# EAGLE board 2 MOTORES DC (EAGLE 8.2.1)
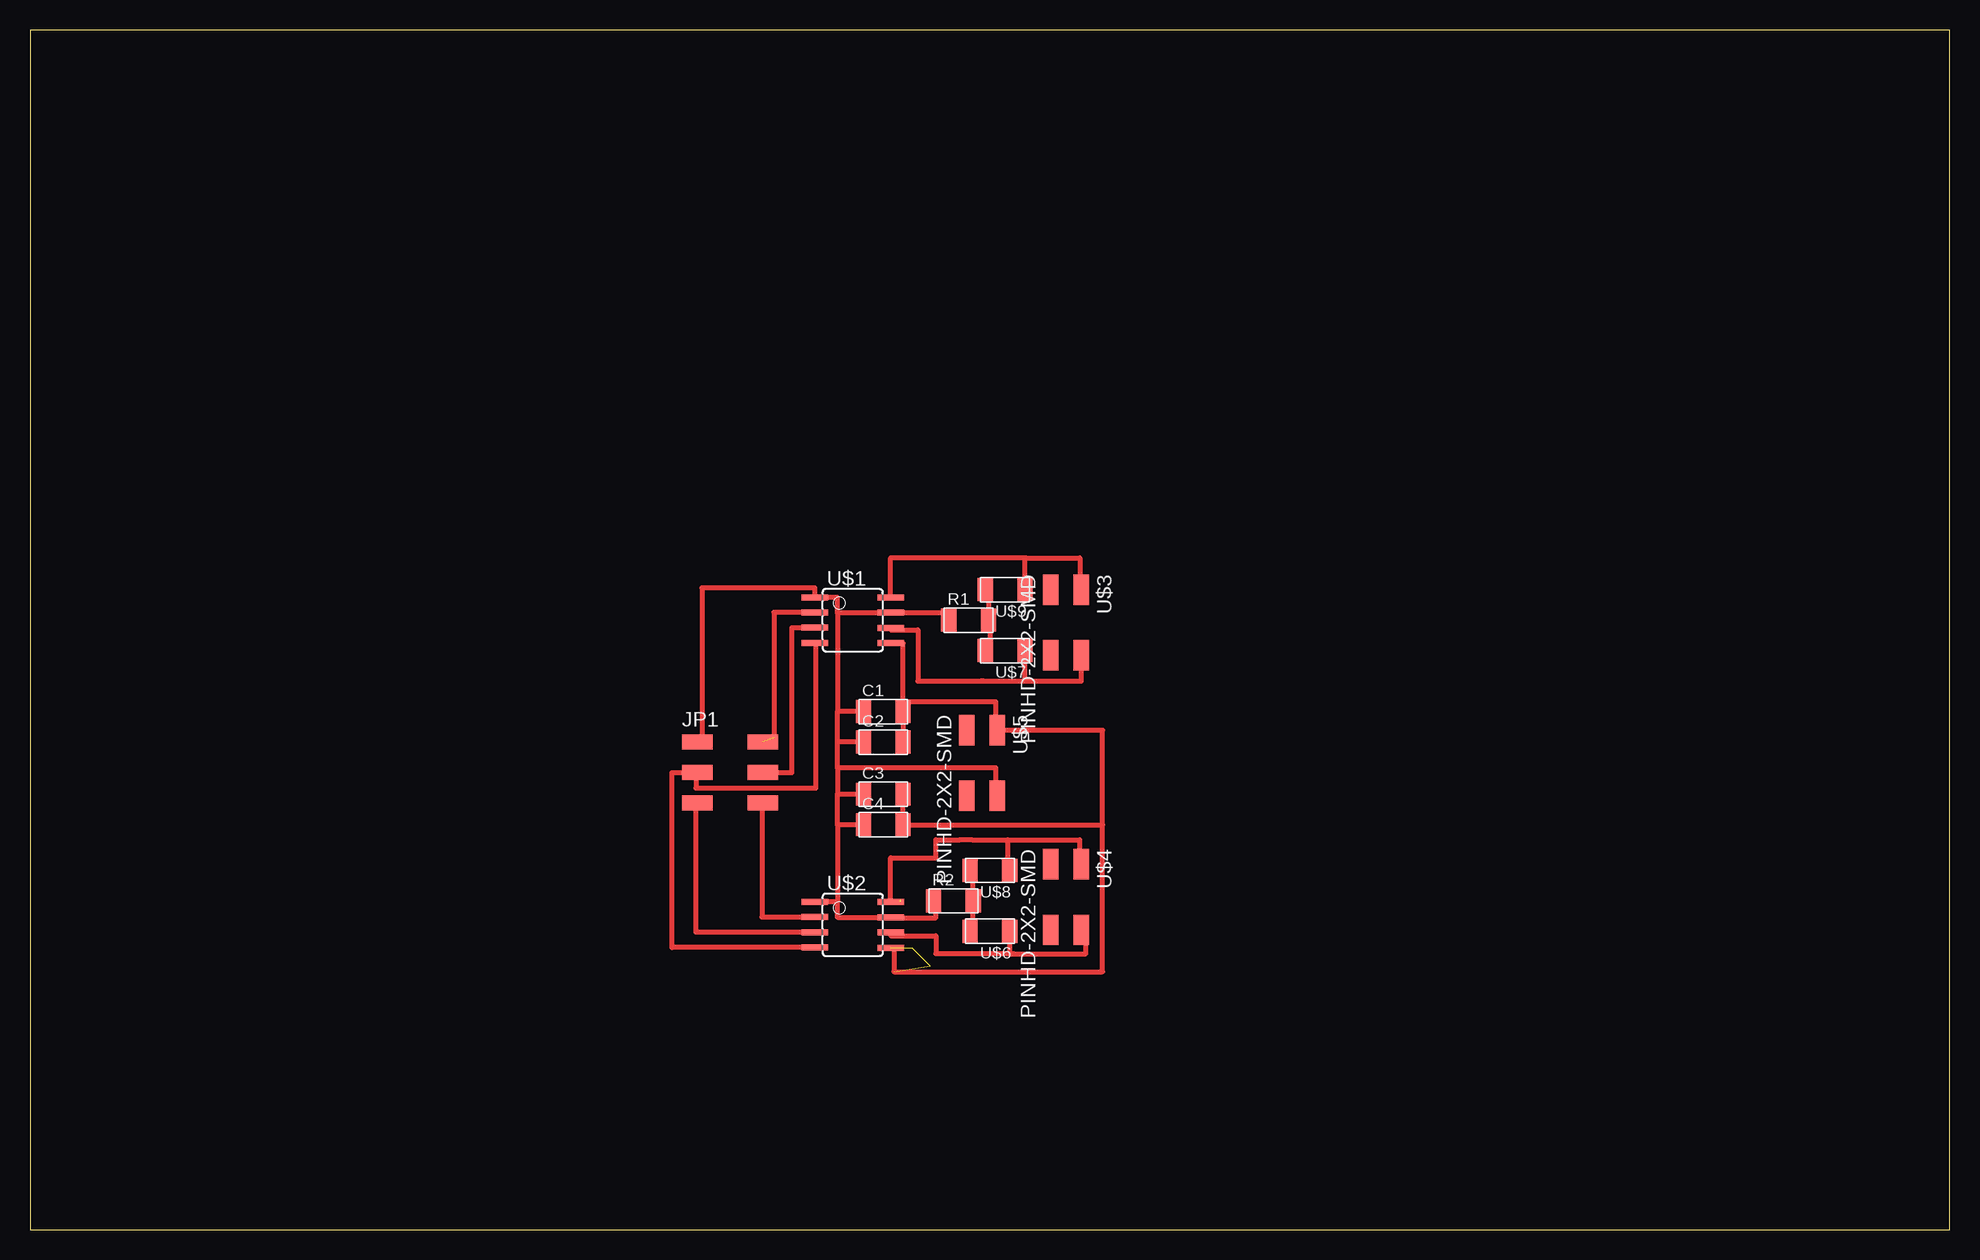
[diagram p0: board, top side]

Size 160 x 100 mm. Coordinates in mm from the lower left corner, seen from the top.
Outline: 0,0 160,0 160,100 0,100 0,0
Copper layers (1*16): Top 0.035mm / dielectric 1.5mm / Bottom 0.035mm
Design rules "default *": minimum track width 10mil, minimum drill 24mil, track to track 16mil, track to pad 16mil, pad to pad 16mil, via to via 16mil, smd to smd 16mil, copper to edge 40mil, drill to drill 8mil, minimum pad ring 10mil, minimum via ring 8mil, stop-mask expansion 4mil, vias tented up to drill 0mil, thermal gap 10mil

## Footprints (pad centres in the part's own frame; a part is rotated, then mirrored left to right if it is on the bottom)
C1206FAB = smd 1.27 x 1.905: 1 -1.651,0; 2 1.651,0
2X03SMD = smd 2.54 x 1.27: 1 -2.54,2.54; 2 2.92,2.54; 3 -2.54,0; 4 2.92,0; 5 -2.54,-2.54; 6 2.92,-2.54
R1206FAB = smd 1.27 x 1.905: 1 -1.651,0; 2 1.651,0
SOIC8 = smd 0.5 x 2.2: 1 -1.905,-3.154; 2 -0.645,-3.154; 3 0.625,-3.154; 4 1.895,-3.154; 5 1.905,3.154; 6 0.635,3.154; 7 -0.635,3.154; 8 -1.905,3.154
2X02SMD = smd 2.54 x 1.27: 1 -2.54,1.27; 2 2.92,1.27; 3 -2.54,-1.27; 4 2.92,-1.27
LED1206FAB = smd 1.27 x 1.905: 1 -1.651,0; 2 1.651,0

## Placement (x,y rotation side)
C1  [C1206FAB]  71.12,43.18 0 top
C2  [C1206FAB]  71.12,40.64 0 top
C3  [C1206FAB]  71.12,36.29 0 top
C4  [C1206FAB]  71.12,33.75 0 top
JP1  [2X03SMD]  58.15,38.1 0 top
R1  [R1206FAB]  78.24,50.8 0 top
R2  [R1206FAB]  76.97,27.4 0 top
U$1  A4953-H-BRIDGE-MOTOR-DRIVER  [SOIC8]  68.58,50.8 270 top
U$2  A4953-H-BRIDGE-MOTOR-DRIVER  [SOIC8]  68.58,25.4 270 top
U$3  PINHD-2X2-SMD  [2X02SMD]  86.36,50.8 270 top
U$4  PINHD-2X2-SMD  [2X02SMD]  86.36,27.9 270 top
U$5  PINHD-2X2-SMD  [2X02SMD]  79.36,39.1 270 top
U$6  LEDFAB1206  [LED1206FAB]  80.01,24.86 180 top
U$7  LEDFAB1206  [LED1206FAB]  81.28,48.26 180 top
U$8  LEDFAB1206  [LED1206FAB]  80.01,29.94 180 top
U$9  LEDFAB1206  [LED1206FAB]  81.28,53.34 180 top

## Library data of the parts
C1-C4 JP1 R1 R2 U$1-U$9 = fab (1)

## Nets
N$1: JP1.2 U$1.2
N$2: JP1.4 U$1.3
N$3: C1.1 C2.1 C3.1 C4.1 JP1.1 R1.1 R2.1 U$1.1 U$1.7 U$2.1 U$2.7 U$5.2
N$4: JP1.6 U$2.2
N$5: JP1.5 U$2.3
N$6: JP1.3 U$1.4 U$2.4
N$7: U$1.8 U$3.1 U$9.1
N$8: U$1.6 U$3.2 U$7.1
N$9: U$2.8 U$4.1 U$8.1
N$10: U$2.6 U$4.2 U$6.1
N$11: C1.2 C2.2 C3.2 C4.2 U$1.5 U$2.5 U$5.1
N$13: R2.2 U$6.2 U$8.2
N$14: R1.2 U$7.2 U$9.2

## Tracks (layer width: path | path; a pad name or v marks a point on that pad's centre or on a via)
N$1  (1 unrouted)
  Top 0.406: U$1.2 62,51.45 62,41
N$2
  Top 0.406: U$1.3 63.5,50.17 63.5,38.1 JP1.4
N$3
  Top 0.406: 67.31,27.3 U$2.1 | 67.31,40.64 67.31,43.18 | 67.31,38.5 67.31,40.64 | 67.31,38.5 67.31,36.29 | 67.31,51.44 67.31,43.18 | 67.31,51.44 67.31,52.7 U$1.1 65.43,53.5 56,53.5 56,40.64 JP1.1 | 67.31,33.75 67.31,36.29 | 67.31,33.75 67.31,27.3 | 67.31,27.3 67.31,26.04 U$2.7 71.73,26 75.5,26 75.5,27.4 R2.1 | C3.1 67.31,36.29 | C4.1 67.31,33.75 | C1.1 67.31,43.18 | C2.1 67.31,40.64 | 67.31,51.44 U$1.7 76.59,51.44 R1.1 | U$5.2 80.5,36.18 80.5,38.5 67.31,38.5
N$4
  Top 0.406: U$2.2 61,26.05 61,35.56 JP1.6
N$5
  Top 0.406: JP1.5 55.5,35.56 55.5,24.77 U$2.3
N$6
  Top 0.406: U$2.4 53.5,23.5 53.5,38.1 JP1.3 55.5,37.99 55.5,36.8 65.5,36.8 65.5,48.91 U$1.4
N$7
  Top 0.406: U$1.8 71.73,56 83,56 | U$3.1 87.5,53.34 87.5,56 83,56 | U$9.1 82.93,56 83,56
N$8
  Top 0.406: 82.93,45.72 U$7.1 | 82.93,45.72 87.63,45.72 U$3.2 | 79.5,45.72 79.22,45.72 | 79.5,45.72 82.93,45.72 | U$1.6 71.73,50 74,50 74,45.72 79.5,45.72
N$9  (1 unrouted)
  Top 0.406: 81.28,29.94 U$8.1 81.5,29.94 81.5,32.5 | 72.5,27.3 U$2.8 71.73,31 75.5,31 75.5,32.5 77.5,32.5 78.5,32.5 81.5,32.5 | 87.5,29.94 U$4.1 87.5,30.57 87.5,32.5 81.5,32.5
N$10
  Top 0.406: U$2.6 71.73,24.5 75.5,24.5 75.5,23 82,23 | 82,23 88,23 88,24.98 U$4.2 | U$6.1 81.66,23 82,23
N$11  (3 unrouted)
  Top 0.406: 89.4,33.75 89.4,21.5 72,21.5 72,23.5 | 72.39,23.5 U$2.5 | C2.2 C1.2 72.77,44 | U$1.5 72.77,48.9 72.77,44 | C3.2 C4.2 89.4,33.75 | 72.77,44 80.5,44 80.5,41.64 U$5.1 89.4,41.64 89.4,33.75
N$13
  Top 0.406: U$8.2 78.62,29.94 R2.2 78.62,24.86 U$6.2
N$14
  Top 0.406: U$9.2 79.89,53.34 R1.2 80,50.8 80,47.5 79.63,47.5 U$7.2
